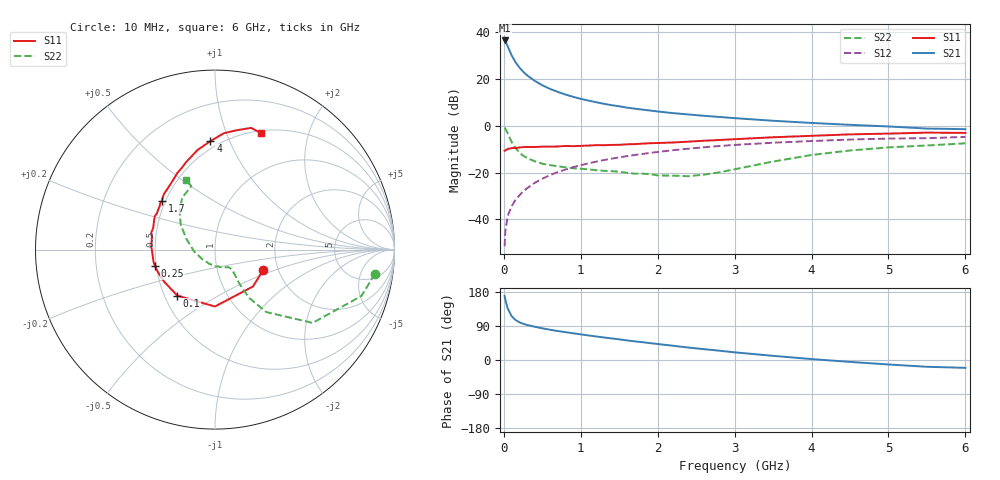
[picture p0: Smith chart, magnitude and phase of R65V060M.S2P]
! SIEMENS Small Signal Semiconductors
! BFR193
! Si NPN RF Bipolar Junction Transistor in SOT23
! VCE = 5 V  IC = 60 mA
! Common Emitter S-Parameters:  May  1996
# GHz  S  MA  R  50
!  f  S11  S21  S12  S22
! GHz  MAG  ANG  MAG  ANG  MAG  ANG  MAG  ANG
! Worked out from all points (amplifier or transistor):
!   36 points, 10 MHz to 6 GHz, reference 50 ohm
!   highest |S21| = 36.3 dB at 10 MHz (marker M1)
!   |S21| within 3 dB of that: start of sweep to 57.01 MHz
!   unconditionally stable (mu >= 1): 375.1 MHz to 1.88 GHz; 1.952 GHz to 2.036 GHz
!   at 250 MHz: K = 0.96, MSG = 25.5 dB, |S12| = -28.1 dB
!   at 1.4 GHz: K = 1.02, MAG = 10.5 dB, |S12| = -14.1 dB
!   at 6 GHz: K = 0.95, MSG = 1.7 dB, |S12| = -4.8 dB
!   S11 on the Smith chart (normalised r, x): 10 MHz: 1.67, -0.42; 100 MHz: 0.58, -0.33; 250 MHz: 0.49, -0.10; 1.7 GHz: 0.48, +0.31; 4 GHz: 0.45, +0.85; 6 GHz: 0.53, +1.34
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0.01  0.2913 -23.2  65.04 169.0  0.0027 83.5  0.9016 -8.6
0.02  0.2951 -44.1  62.27 158.7  0.0057 79.6  0.8555 -17.6
0.05  0.3171 -90.1  48.94 136.0  0.0119 69.4  0.6801 -36.9
0.1  0.3313 -129.4  31.67 116.0  0.019 69.6  0.4506 -50.6
0.15  0.335 -147.6  22.59 105.8  0.026 70.9  0.3348 -54.5
0.2  0.3405 -157.2  17.44 99.8  0.0324 72.9  0.271 -54.8
0.25  0.3479 -164.5  14.09 95.6  0.0393 73.5  0.2292 -54.2
0.3  0.3494 -169.3  11.85 92.5  0.046 74.8  0.2053 -53.3
0.4  0.3497 -177.0  9.008 87.9  0.06 74.8  0.1738 -51.4
0.5  0.3551 177.7  7.215 83.6  0.0738 74.6  0.1543 -50.2
0.6  0.3562 173.2  6.056 79.9  0.0881 73.9  0.1438 -50.0
0.7  0.3586 168.8  5.223 76.5  0.1017 73.1  0.1364 -50.6
0.8  0.3676 165.0  4.584 73.5  0.1158 71.8  0.1291 -51.6
1.1  0.3753 155.0  3.405 64.8  0.1569 68.0  0.117 -57.7
1.4  0.3875 144.8  2.718 57.0  0.197 63.7  0.1072 -66.4
1.7  0.4025 137.2  2.293 49.2  0.2362 59.4  0.0946 -79.4
2.2  0.4363 125.7  1.841 37.6  0.299 51.7  0.0857 -111.5
3.5  0.5637 99.9  1.267 11.0  0.4313 31.2  0.1713 159.1
4  0.605 92.4  1.138 2.4  0.4691 24.1  0.2362 144.0
4.5  0.65 85.7  1.038 -5.0  0.5033 17.1  0.2949 132.0
5.5  0.7072 73.5  0.864 -17.9  0.5394 3.4  0.3769 110.4
6  0.6984 68.3  0.839 -20.7  0.5732 -0.5  0.4188 112.6
